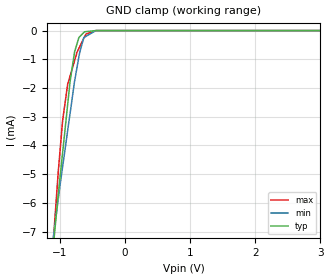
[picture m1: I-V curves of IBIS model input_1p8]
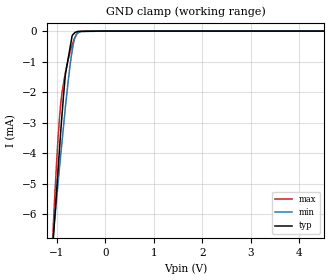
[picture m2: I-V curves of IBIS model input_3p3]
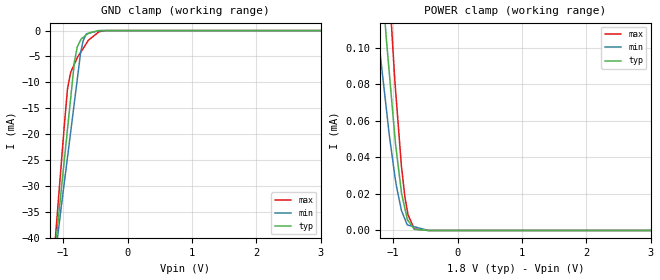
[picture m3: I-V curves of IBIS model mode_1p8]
|Texas Instruments Incorporated
| 93dB SNR Low-Power Stereo DAC with HP Amplifier (S/W Control)
| Marketing part#   Digital Voltage Range   Package-type   #pins
| PCM1774RGPR   1.71V - 3.6V   QFN   20
| PCM1774RGPRG4   1.71V - 3.6V   QFN   20
| PCM1774RGPT   1.71V - 3.6V   QFN   20
| PCM1774RGPTG4   1.71V - 3.6V   QFN   20
[IBIS Ver]   3.2
[File name]   pcm1774.ibs
[File Rev]   1.0
[Date]   10/13/2011
[Source]
| Texas Instruments Incorporated.
| Analog-eLab Design Center, HPA
| 12500 TI Blvd
| Dallas, TX -75243
| e-mail: elab_scm_ibis@list.ti.com
[Notes]   Revision History:
| Rev 1.0: 10/13/2011
| - Initial version of the model
| - Model generated from simulations in SPECTRE
| - Model matched to SPICE simulation
| - C_comp although listed in numerical order of value are
|   obtained from varying PVT conditions. For PVT conditions for
|   each specific value refer the buffer description under
|   respective [Model]. IBIS model user is responsible for using
|   appropriate C_comp to simulate for Signal Integrity.
| - Model names with a trailing _1p8 contains the model for
|   1.8V [1.71V and 1.89V].Model names with a trailing _3p3
|   contains the model for 3.3V [3.0V and 3.6V].
[Disclaimer]
| This model is designed as an aid for customers of Texas Instruments.
| TI and its licensors and suppliers make no warranties, either expressed
| or implied, with respect to this  model, including the warranties of
| merchantability or fitness for a particular purpose. The model is
| provided solely on an "as is" basis. The entire risk as to its quality
| and performance is with the customer.
[Copyright]
 (C) Copyright 2011 Texas Instruments Incorporated.All rights reserved.
|   PCM1774
[Component]   PCM1774
[Manufacturer]   TI
[Package]   |20 QFN   -  RGP package
|   typ   min   max
R_pkg   0.06398   0.05933   0.07397
L_pkg   1.05005nH   0.97320nH   1.21841nH
C_pkg   0.14726pF   0.13386pF   0.15889pF
[Pin]  signal_name   model_name   R_pin   L_pin   C_pin
1   MODE   MODE   0.06148   1.01388nH  0.13812pF
2   MS/ADR   INPUT   0.05960   0.97699nH  0.15085pF
3   MD/SDA   IO   0.05980   0.97952nH  0.15188pF
4   MC/SCL   INPUT   0.06692   1.09860nH  0.15889pF
5   DIN   INPUT   0.06522   1.07683nH  0.14050pF
6   VIO   POWER   0.03197   0.76301nH  0.16601pF
7   VDD   POWER   0.05985   0.97820nH  0.15321pF
8   DGND   GND   0.03041   0.69450nH  0.18093pF
9   SCKI   INPUT   0.06289   1.02576nH  0.15706pF
10   BCK   IO   0.07292   1.20130nH  0.15166pF
11   LRCK   IO   0.07397   1.21841nH  0.14811pF
12   PGND   GND   0.08019   1.32158nH  0.17249pF
13   VPA   POWER   0.06219   1.01171nH  0.15562pF
14   HPOR/LOR   TERM   0.06393   1.04112nH  0.15619pF
15   HPOL/LOL   TERM   0.06612   1.08440nH  0.14204pF
16   VCOM   TERM   0.06004   0.98569nH  0.13677pF
17   AGND   GND   0.06106   0.99863nH  0.15296pF
18   VCC   POWER   0.06247   1.02186nH  0.15215pF
19   AIN1R   TERM   0.05956   0.97320nH  0.14850pF
20   AIN1L   TERM   0.05933   0.97497nH  0.13386pF
|   Model Selectors
[Model Selector] INPUT
input_1p8  1.8V digital input
input_3p3  3.3V digital input
[Model Selector] MODE
mode_1p8  1.8V digital input
mode_3p3  3.3V digital input
[Model Selector] IO
io_1p8  1.8V digital I/O
io_3p3  3.3V digital I/O
[Model Selector] TERM
term_1-8V  1.8V nominal termination
term_3-3V  3.3V nominal termination
[Model] term_1-8V
Model_type Terminator
C_comp   1.0e-20F  1.0e-20F  1.0e-20F
|   typ   min   max
[Voltage Range]   1.8V   1.71V   1.89V
[POWER Clamp Reference]   1.8V   1.71V   1.89V
[GND Clamp Reference]   0V   0V   0V
|Ambient Temperature   25   85   -40
|Junction Temperature
[Temperature Range]   26   86   -40
[Model] term_3-3V
Model_type Terminator
C_comp   1.0e-20F  1.0e-20F  1.0e-20F
|   typ   min   max
[Voltage Range]   3.3V   3.0V   3.6V
[POWER Clamp Reference]   3.3V   3.0V   3.6V
[GND Clamp Reference]   0V   0V   0V
|Ambient Temperature   25   85   -40
|Junction Temperature
[Temperature Range]   26   86   -40
| Models and submodels in the file (8): input_1p8 (Input), input_3p3 (Input), mode_1p8 (Input), mode_3p3 (Input), io_1p8 (I/O), io_3p3 (I/O), term_1-8V (Terminator), term_3-3V (Terminator)
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|   input_1p8 Model
[Model]   input_1p8
Model_type   Input
Vinl = 0.54
Vinh = 1.26
|   typ   min   max
|   (nom PVT)   (fast PVT)   (slow PVT)
C_comp   1.824e-13   5.668e-14   2.684e-13
| Where nom  PVT is Nominal Process, 1.8V, 26C
|   Fast PVT is Strong Process,  1.89V, -40C
|   Slow PVT is Weak Process,   1.71V, 86C
[Model Spec]
|Subparameter   typ   min   max
Vinh   1.26   1.197   1.323
Vinl   0.54   0.513   0.567
[Voltage Range]   1.8   1.71   1.89
|Ambient Temperature   25   85   -40
|Junction Temperature
[Temperature Range]   26   86   -40
[Power Clamp Reference]   1.8   1.71   1.89
[GND Clamp Reference]   0   0   0
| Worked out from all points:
|   GND clamp passes 1 mA (typ) near -0.79 V on its own axis
[GND Clamp]
|   Voltage   I(typ)   I(min)   I(max)
-1.8V     -24.34mA   -19.47mA   -31.1mA
-1.11V    -7.726mA   -7.352mA   -7.592mA
-1.03V    -5.786mA   -5.938mA   -5.043mA
-957.1mV  -4.216mA   -4.716mA   -3.105mA
-881.5mV  -2.58mA    -3.489mA   -1.874mA
-842.4mV  -1.748mA   -2.855mA   -1.571mA
-774mV    -735.3uA   -1.751mA   -1.04mA
-698.8mV  -218.3uA   -786.8uA   -574.9uA
-622.8mV  -41.88uA   -230.8uA   -222.4uA
-601.7mV  -36.82uA   -202.9uA   -124.7uA
-449.1mV  -344nA     -1.004uA   -1.889uA
3.6V      0A         0A         0A
[POWER Clamp]
|   Voltage   I(typ)   I(min)   I(max)
-1.8V     0A         0A         0A
3.6V      0A         0A         0A
|   input_3p3 Model
[Model]   input_3p3
Model_type   Input
Vinl = 0.99
Vinh = 2.31
|   typ   min   max
|   (nom PVT)   (fast PVT)   (slow PVT)
C_comp   1.824e-13   5.668e-14   2.582e-13
| Where nom  PVT is Nominal Process, 3.3V, 26C
|   Fast PVT is Strong Process,  3.6V, -40C
|   Slow PVT is Weak Process,   3V, 86C
[Model Spec]
|Subparameter   typ   min   max
Vinh   2.31   2.1   2.52
Vinl   0.99   0.9   1.08
[Voltage Range]   3.3   3   3.6
|Ambient Temperature   25   85   -40
|Junction Temperature
[Temperature Range]   26   86   -40
[Power Clamp Reference]   3.3   3   3.6
[GND Clamp Reference]   0   0   0
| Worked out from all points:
|   GND clamp passes 1 mA (typ) near -0.78 V on its own axis
[GND Clamp]
|   Voltage   I(typ)   I(min)   I(max)
-3.3V     -60.52mA   -45.86mA   -82.36mA
-1.089V   -7.173mA   -6.948mA   -6.84mA
-1.056V   -6.377mA   -6.374mA   -5.794mA
-978mV    -4.592mA   -5.015mA   -3.561mA
-942mV    -3.769mA   -4.402mA   -2.752mA
-895.2mV  -2.752mA   -3.637mA   -2.012mA
-825mV    -1.424mA   -2.496mA   -1.357mA
-686.4mV  -156.2uA   -652.2uA   -454uA
-627mV    -44.46uA   -210.4uA   -209.9uA
-537mV    -9.471uA   -16.27uA   -37.49uA
-391.2mV  -6.342uA   -10.74uA   -26.9nA
6.6V      0A         0A         0A
[POWER Clamp]
|   Voltage   I(typ)   I(min)   I(max)
-3.3V     0A         0A         0A
6.6V      0A         0A         0A
|   mode_1p8 Model
[Model]   mode_1p8
Model_type   Input
Vinl = 0.54
Vinh = 1.26
|   typ   min   max
|   (nom PVT)   (fast PVT)   (slow PVT)
C_comp   8.959e-13   8.859e-13   9.027e-13
| Where nom  PVT is Nominal Process, 1.8V, 26C
|   Fast PVT is Strong Process,  1.89V, -40C
|   Slow PVT is Weak Process,   1.71V, 86C
[Model Spec]
|Subparameter   typ   min   max
Vinh   1.26   1.197   1.323
Vinl   0.54   0.513   0.567
[Voltage Range]   1.8   1.71   1.89
|Ambient Temperature   25   85   -40
|Junction Temperature
[Temperature Range]   26   86   -40
[Power Clamp Reference]   1.8   1.71   1.89
[GND Clamp Reference]   0   0   0
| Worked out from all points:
|   GND clamp passes 1 mA (typ) near -0.66 V on its own axis
[GND Clamp]
|   Voltage   I(typ)   I(min)   I(max)
-1.8V     -127.5mA   -112.9mA   -149.8mA
-1.097V   -39.15mA   -40.96mA   -36.35mA
-1.053V   -33.64mA   -36.47mA   -29.46mA
-930.6mV  -18.82mA   -24.29mA   -11.14mA
-883.3mV  -13.1mA    -19.6mA    -8.07mA
-826.2mV  -6.179mA   -13.94mA   -6.489mA
-783mV    -3.303mA   -9.659mA   -5.295mA
-727.8mV  -1.812mA   -4.252mA   -4.203mA
-688.5mV  -1.314mA   -1.925mA   -3.439mA
-640.6mV  -838.9uA   -652.1uA   -2.509mA
-346.6mV  -611nA     0A         -18.36uA
3.6V      0A         0A         0A
[POWER Clamp]
|   Voltage   I(typ)   I(min)   I(max)
-1.8V     467.8uA    288.4uA    734.1uA
-1.334V   212.1uA    144uA      323.3uA
-1.202V   149.9uA    96.6uA     229.6uA
-1.131V   116.7uA    74.47uA    180.7uA
-1.107V   105.4uA    66.96uA    164.7uA
-1.05V    82.17uA    49.66uA    126.3uA
-963mV    47.27uA    27.32uA    77.07uA
-872mV    21.06uA    11.07uA    35.43uA
-819.1mV  12.36uA    6.36uA     18.83uA
-770mV    5.478uA    2.927uA    8.686uA
-671.4mV  620.3nA    2.028uA    816.9nA
3.6V      0A         0A         0A
